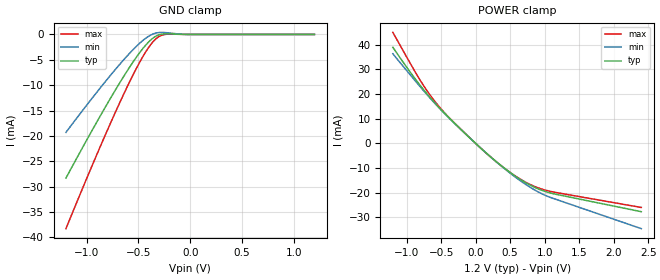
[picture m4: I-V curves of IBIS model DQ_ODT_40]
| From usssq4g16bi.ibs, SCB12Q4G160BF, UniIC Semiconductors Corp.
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|   Model DQ_ODT_40
[Model] DQ_ODT_40
Model_type Input
Polarity   Non-Inverting
Enable   Active-High
Vinl =  8.300E-01
Vinh =  9.700E-01
C_comp   7.827E-13   7.748E-13   8.022E-13
C_comp_power_clamp   2.050E-13   1.847E-13   2.346E-13
C_comp_gnd_clamp   5.777E-13   5.676E-13   5.901E-13
[Model Spec]
Vinh   9.700E-01   9.250E-01   1.015E+00
Vinl   8.300E-01   7.850E-01   8.750E-01
[Temperature Range]   45.000   95.000   -40.0
[Voltage Range]   1.200E+00   1.140E+00   1.260E+00
[C Comp Corner]
C_comp_power_clamp   2.050E-13   1.847E-13   2.346E-13
C_comp_gnd_clamp   5.777E-13   5.901E-13   5.676E-13
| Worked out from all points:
|   GND clamp passes 1 mA (typ) near -0.38 V on its own axis
|   POWER clamp passes 1 mA (typ) near -0.04 V on its own axis
[GND_clamp]
|Voltage   I(typ)   I(min)   I(max)
-1.2V     -28.31mA   -19.3mA    -38.28mA
-875mV    -16.3mA    -10.7mA    -22.4mA
-750mV    -11.89mA   -7.566mA   -16.58mA
-625mV    -7.714mA   -4.602mA   -11.03mA
-525mV    -4.633mA   -2.451mA   -6.902mA
-450mV    -2.592mA   -1.071mA   -4.123mA
-375mV    -973.6uA   -56.79uA   -1.832mA
-325mV    -274uA     305uA      -753.5uA
-275mV    59.15uA    401.4uA    -154.4uA
-200mV    121.1uA    281.3uA    62.53uA
-25mV     0A         0A         0A
1.2V      0A         0A         0A
[POWER_clamp]
|Voltage   I(typ)   I(min)   I(max)
-1.2V     39.02mA    36.37mA    45.05mA
-975mV    29.96mA    28.73mA    33.85mA
-800mV    23.42mA    22.89mA    25.47mA
-675mV    19.16mA    18.84mA    20.17mA
-525mV    14.42mA    14.27mA    14.78mA
-350mV    9.362mA    9.33mA     9.476mA
75mV      -1.94mA    -1.938mA   -1.965mA
300mV     -7.432mA   -7.509mA   -7.479mA
500mV     -11.81mA   -12.08mA   -11.79mA
775mV     -16.73mA   -17.55mA   -16.47mA
1.025V    -19.66mA   -21.27mA   -19.07mA
2.4V      -27.71mA   -34.59mA   -26mA
